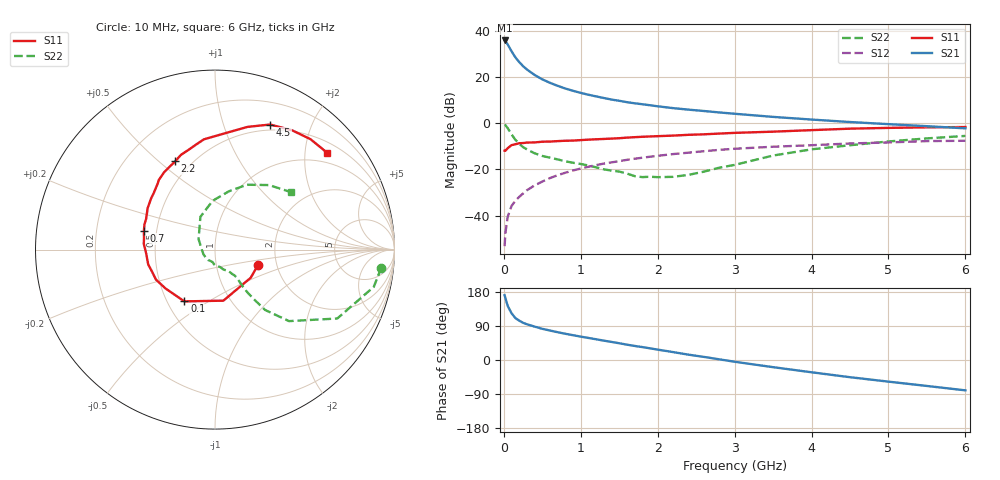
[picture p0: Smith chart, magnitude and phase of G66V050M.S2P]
! SIEMENS Small Signal Semiconductors
! BFG193
! Si NPN RF Bipolar Junction Transistor in SOT223
! VCE = 6 V  IC = 50 mA
! Common Emitter S-Parameters:  August  1996
# GHz  S  MA  R  50
!  f  S11  S21  S12  S22
! GHz  MAG  ANG  MAG  ANG  MAG  ANG  MAG  ANG
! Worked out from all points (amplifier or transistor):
!   36 points, 10 MHz to 6 GHz, reference 50 ohm
!   highest |S21| = 35.8 dB at 10 MHz (marker M1)
!   |S21| within 3 dB of that: start of sweep to 71.75 MHz
!   unconditionally stable (mu >= 1): 466.9 MHz to 2.414 GHz
!   at 250 MHz: K = 0.91, MSG = 27.5 dB, |S12| = -30.4 dB
!   at 1.4 GHz: K = 1.04, MAG = 12.3 dB, |S12| = -16.9 dB
!   at 6 GHz: K = 0.89, MSG = 2.7 dB, |S12| = -7.6 dB
!   S11 on the Smith chart (normalised r, x): 10 MHz: 1.60, -0.29; 100 MHz: 0.61, -0.40; 700 MHz: 0.42, +0.11; 2.2 GHz: 0.41, +0.57; 4.5 GHz: 0.44, +1.44; 6 GHz: 0.74, +2.51
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0.01  0.255 -19.4  61.34 171.0  0.0022 96.0  0.9319 -6.2
0.02  0.2534 -38.3  59.07 163.6  0.0042 82.0  0.9087 -13.2
0.05  0.2883 -80.7  50.27 143.0  0.0095 71.3  0.782 -29.4
0.1  0.3352 -120.6  35.9 123.3  0.0163 68.6  0.5736 -44.0
0.15  0.3507 -141.9  26.47 110.7  0.0211 66.7  0.4374 -50.3
0.2  0.369 -153.1  20.91 103.8  0.0256 67.5  0.36 -51.7
0.25  0.372 -161.2  17.09 98.2  0.0302 68.5  0.3038 -52.8
0.3  0.3812 -167.4  14.46 94.3  0.0356 69.0  0.2715 -53.1
0.4  0.384 -176.6  11.02 88.1  0.0452 69.0  0.2236 -52.6
0.5  0.3981 175.3  8.858 82.3  0.0548 68.3  0.1958 -52.2
0.6  0.4006 170.8  7.443 77.8  0.0651 67.5  0.1798 -53.0
0.7  0.4098 165.3  6.415 73.3  0.0752 66.5  0.1649 -55.0
0.9  0.4205 155.8  5.006 65.4  0.0952 62.5  0.1395 -58.0
1.1  0.4409 148.3  4.118 58.2  0.1146 59.2  0.1218 -66.5
1.3  0.4565 141.2  3.498 51.1  0.134 55.2  0.1007 -73.9
1.6  0.4873 130.9  2.848 40.5  0.1614 48.4  0.0816 -94.0
2.2  0.5393 114.3  2.116 20.9  0.2149 34.9  0.0693 -157.1
2.8  0.5966 99.8  1.708 1.8  0.2652 21.0  0.1091 147.3
3.5  0.6559 83.9  1.368 -18.9  0.3099 3.8  0.1999 114.0
4.5  0.7616 66.2  1.059 -45.4  0.3643 -16.1  0.3338 76.6
5.5  0.8134 49.1  0.861 -68.5  0.4103 -39.4  0.4693 50.0
6  0.8258 40.7  0.774 -80.1  0.4166 -52.8  0.5306 37.1
